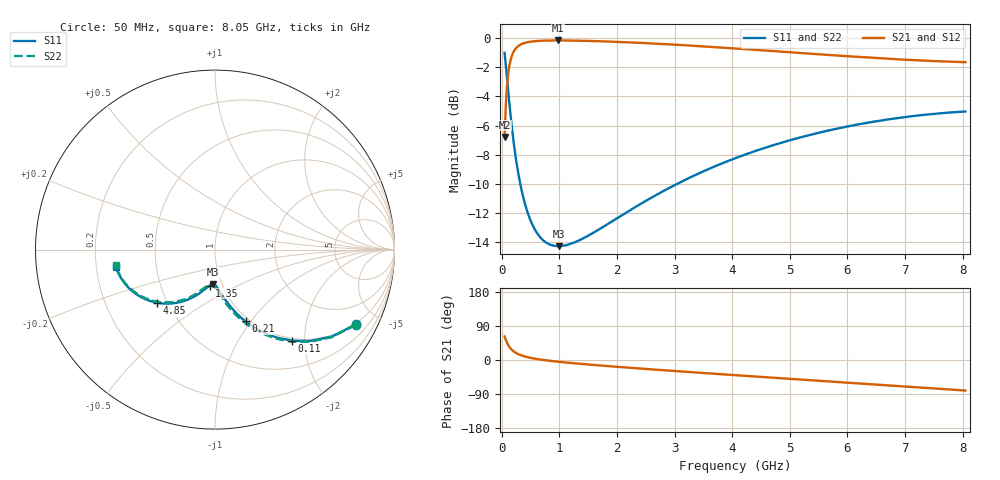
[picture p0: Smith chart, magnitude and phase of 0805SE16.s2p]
! AVX Thin Film Operation		Date: August 2001
! Description: Accu-P® Series, Thin Film, SMD, RF Capacitor
! Part Number: 08055K160FBT
! 50 MHz  -  8.05 GHz
! Serial Measurements
# mhz S db R 50
!	S11		S21		S12		S22
!	dB	Phase	dB	Phase	dB	Phase	dB	Phase
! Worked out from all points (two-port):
!   401 points, 50 MHz to 8.05 GHz, reference 50 ohm
!   highest |S21| = -0.17 dB at 970 MHz (marker M1); lowest = -6.8 dB at 50 MHz (marker M2)
!   |S21| within 3 dB of the highest: 95.22 MHz to end of sweep
!   lowest |S11| = -14.3 dB at 990 MHz (marker M3), VSWR 1.48, Z = 45.5 - j18.3 ohm
!   |S11| at or under -10 dB: 322.1 MHz to 3.042 GHz (2.719 GHz wide, 162 % of centre)
!   |S22| runs from -14.3 to -1.0 dB; largest |S21 - S12| = 0
!   S11 on the Smith chart (normalised r, x): 50 MHz: 0.96, -3.80; 110 MHz: 0.96, -1.74; 210 MHz: 0.96, -0.94; 1.35 GHz: 0.87, -0.36; 4.85 GHz: 0.44, -0.32; 8.05 GHz: 0.28, -0.08
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50  -1.02 -27.9  -6.79 62.0  -6.79 62.0  -1.02 -28.2
70  -1.81 -36.6  -4.69 53.2  -4.69 53.2  -1.81 -37.0
110  -3.54 -49.7  -2.54 40.0  -2.54 40.0  -3.54 -50.4
150  -5.17 -58.5  -1.58 31.1  -1.58 31.1  -5.17 -59.4
170  -5.91 -61.8  -1.29 27.7  -1.29 27.7  -5.91 -62.8
210  -7.24 -67.0  -0.91 22.4  -0.91 22.4  -7.24 -68.2
270  -8.87 -72.4  -0.61 16.8  -0.61 16.8  -8.87 -74.0
330  -10.16 -76.3  -0.44 12.8  -0.44 12.8  -10.16 -78.1
410  -11.46 -80.0  -0.33 8.9  -0.33 8.9  -11.46 -82.1
510  -12.60 -83.3  -0.25 5.4  -0.25 5.4  -12.60 -85.8
710  -13.83 -88.2  -0.19 0.3  -0.19 0.3  -13.83 -91.0
970  -14.26 -92.8  -0.17 -4.4  -0.17 -4.4  -14.26 -95.8
990  -14.26 -93.1  -0.17 -4.7  -0.17 -4.7  -14.26 -96.1
1350  -13.85 -98.4  -0.19 -9.9  -0.19 -9.9  -13.85 -101.2
1390  -13.78 -98.9  -0.19 -10.4  -0.19 -10.4  -13.78 -101.8
2010  -12.33 -106.7  -0.27 -18.0  -0.27 -18.0  -12.33 -109.1
2730  -10.65 -115.0  -0.40 -26.1  -0.40 -26.1  -10.65 -117.0
4050  -8.24 -129.2  -0.71 -40.0  -0.71 -40.0  -8.24 -130.6
4850  -7.18 -137.4  -0.93 -48.2  -0.93 -48.2  -7.18 -138.7
5390  -6.60 -142.9  -1.08 -53.6  -1.08 -53.6  -6.60 -144.1
6730  -5.57 -156.4  -1.43 -67.1  -1.43 -67.1  -5.57 -157.4
8050  -5.04 -169.9  -1.66 -80.6  -1.66 -80.6  -5.04 -170.9
